(* 	
	Program Name: 	ACS_SAMPLE_VELOCITY_MOVES
	Purpose:		Example of a program that runs a series of velocity moves at specified intervals 
	When Executed:	Assuming the cycle rate of the PLC is 10ms, this will execute a given speed for a given number of milliseconds, then start the next velocity
*)
PROGRAM ACS_SAMPLE_VELOCITY_MOVES
VAR_IN_OUT 
	Axis:ACS_DRIVE_TYPE;
END_VAR

VAR_INPUT
	
	Speed1			:REAL;
	Speed2			:REAL;
	Speed3			:REAL;
	AccelDecel		:REAL;
	Force			:REAL;
	TimeInSpeedMS	:UDINT;
END_VAR

VAR
	_readyToRumble		:BOOL;
	_timeMidPoint		:UDINT;
	_currentTimeInMS	:UDINT	:=0;
	_cycleTimeInMS		:UDINT	:=10;
	_currentSpeedIdx	:USINT	:=1;
END_VAR

(* 
	This program contains both the input and output scan and is intented to be a stand alone application
	Remember : The input scan should be one of the first things done in the program.  Then the processing.  
	Then the Output Scan.
	|->Input Scan
	|
	|->Processing (User Code)
	|
	|->Output Scan
*)

//Input Scan Routine
ACS_DRIVE_INPUT_SCAN(Axis:=Axis);

//Processing (User Code)

//Step 1. Initialize the drive
//Velocity moves clear the home bit.  So we are basically looking for faults and enabling the drive if its not enabled.
IF Axis.InputFaultActive < 1 THEN

	//If we are not enabled, then enable
	IF Axis.InputStatusDriveEnabled < 1 THEN
		ACS_CMD_ENABLE(Axis:=Axis);
	END_IF
	
END_IF

//Step 2. Determine if we are Ready To Rumble (motion is possible)
_readyToRumble := (Axis.InputStatusDriveEnabled AND NOT Axis.InputFaultActive);	
_timeMidPoint  :=  TimeInSpeedMS / 2; 

//Step 4. Run program based on extend or retracted state
IF _readyToRumble THEN
	
	_currentTimeInMS := _currentTimeInMS + _cycleTimeInMS;
	
	IF _currentTimeInMS > TimeInSpeedMS THEN
		_currentTimeInMS := 0;
		_currentSpeedIdx := _currentSpeedIdx + 1;
		IF _currentSpeedIdx > 3 THEN
			_currentSpeedIdx := 1;
		END_IF
	END_IF
	
	IF _currentSpeedIdx = 1 THEN
		ACS_MOVE_VELOCITY_ROTARY_FORWARD(Axis:=Axis,
			ProfileVelocity := Speed1,
			ProfileAcceleration := AccelDecel,
			ProfileDeceleration := AccelDecel,
			ProfileForce := Force);
	END_IF
	
	IF _currentSpeedIdx = 2 THEN
		ACS_MOVE_VELOCITY_ROTARY_FORWARD(Axis:=Axis,
			ProfileVelocity := Speed2,
			ProfileAcceleration := AccelDecel,
			ProfileDeceleration := AccelDecel,
			ProfileForce := Force);
	END_IF
	
	IF _currentSpeedIdx = 3 THEN
		ACS_MOVE_VELOCITY_ROTARY_FORWARD(Axis:=Axis,
			ProfileVelocity := Speed3,
			ProfileAcceleration := AccelDecel,
			ProfileDeceleration := AccelDecel,
			ProfileForce := Force);
	END_IF
	
	IF _currentTimeInMS < _timeMidPoint THEN
		ACS_CMD_START_MOTION(Axis := Axis);
	ELSE
		ACS_CMD_CLEAR_START_MOTION(Axis := Axis);
	END_IF
	
END_IF

//End processing (User Code)

//Output Scan Routine
ACS_DRIVE_OUTPUT_SCAN(Axis:=Axis);

END_PROGRAM
